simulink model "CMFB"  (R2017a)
settings: Solver=ode113  StartTime=0.0  StopTime=3  RelTol=1e-4  EnableMultiTasking=on
model workspace: external: MAT-File (data not in the file)
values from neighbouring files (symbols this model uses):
  Button = readtable('i_button.csv')    [CMFBoptimizer.m]
  Button_Stiffness = table(x_displacement,stiffness,activation_p,activation_d,activation_midair,damping)    [CMFBoptimizer.m]
  Finger = readtable('i_finger.csv')    [CMFBoptimizer.m]
  finger_start_height = random('norm',Finger.fstart_height,Finger.fstart_height_std)    [CMFBoptimizer.m]
  Finger_Stiffness = readtable('i_finger_stiffness.csv')    [CMFBoptimizer.m]
  Sensory = readtable('i_sensorynoise.csv')    [CMFBoptimizer.m]
undefined symbols (not defined in the file or in its folder): amplitude_ag, amplitude_an, b_penvel, Circle, circle_rad, Contact_Forces_Lib, deg, Extr_Data_Ring, Finite, Force, k_pen, kg, Law, Line, line_depth, line_length, m, max_out, min_out, N, PD, pen_exp, phasedelay_ag, PL, pulsewidth_ag, pulsewidth_an, PW, s, step_finish, step_start, to, vis_len_cirFx, vis_len_linBx, vis_len_linBz, vis_opc, vis_opc_en, window, X, Y, Z
libraries: nesl_utility x40, sm_lib x36, Contact_Forces_Lib x2, fl_lib x2, powerlib_meascontrol x1
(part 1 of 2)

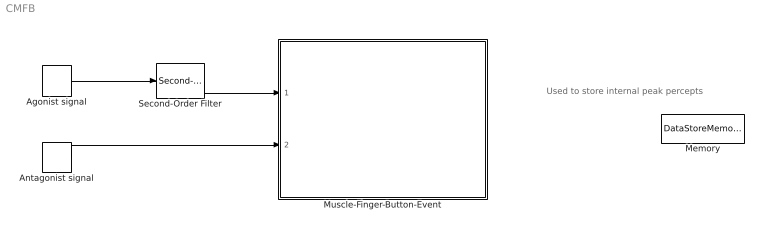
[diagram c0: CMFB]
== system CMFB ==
  note: Used to store internal peak percepts
  Agonist signal : DiscretePulseGenerator  PulseType=Time based  Amplitude=amplitude_ag  Period=window  PulseWidth=pulsewidth_ag  PhaseDelay=phasedelay_ag
  Antagonist signal : DiscretePulseGenerator  PulseType=Time based  Amplitude=amplitude_an  Period=window  PulseWidth=pulsewidth_an
  Memory : DataStoreMemory  DataStoreName=peak_int  ReadBeforeWriteMsg=warning  WriteAfterWriteMsg=warning  WriteAfterReadMsg=warning  InitialValue=0.1  ShowAdditionalParam=off  OutMin=0  OutMax=window
  Muscle-Finger-Button-Event : Subsystem
  Second-Order Filter : powerlib_meascontrol/Filters/Second-Order Filter  FilterType=Lowpass  Fo=4  Zeta=0.9  Ts=0  Initialize=on  Vac_Init="[0,  0,  60]"  Vdc_Init=0  PlotResponse=off  FreqRange=[0, 500, 1]
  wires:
  Antagonist signal/1 -> Muscle-Finger-Button-Event/2(Antagonist Muscle activation signal (0 to 1)1)
  Agonist signal/1 -> Second-Order Filter/1
  Second-Order Filter/1 -> Muscle-Finger-Button-Event/1(Agonist Muscle activation signal (0 to 1))

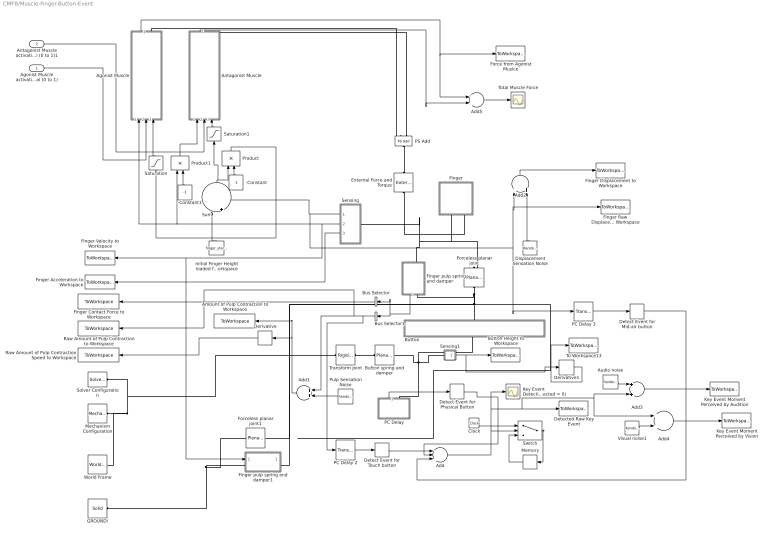
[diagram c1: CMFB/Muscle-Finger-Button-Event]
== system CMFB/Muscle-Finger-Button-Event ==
  Agonist Muscle activation signal (0 to 1) : Inport
  Antagonist Muscle activation signal (0 to 1)1 : Inport  Port=2
  -Constant : Constant  Value=-1
  -Constant1 : Constant  Value=-1
  Add : Sum  Inputs=+++
  Add{1..5} (5 alike) : Sum
  Agonist Muscle : Subsystem
  Amount of Pulp Contraction to Workspace : ToWorkspace  VariableName=pulpcontact  SaveFormat=Timeseries  SampleTime=-1
  Antagonist Muscle : Subsystem
  Audio noise : RandomNumber  Variance=Sensory.a_noise
  Bus Selector : BusSelector  OutputSignals=Normal Force  OutputAsBus=on
  Bus Selector1 : BusSelector  OutputSignals=Penetration  OutputAsBus=on
  Button : Subsystem  Tag=CustomStyle
  Button spring and damper : sm_lib/Joints/Planar Joint  SenseConstraintForce=off  SenseConstraintForceX=off  SenseConstraintForceY=off  SenseConstraintForceZ=off  SenseConstraintTorque=off  SenseConstraintTorqueX=off  SenseConstraintTorqueY=off  SenseConstraintTorqueZ=off  SenseTotalForce=off  SenseTotalForceX=off  SenseTotalForceY=off  SenseTotalForceZ=off  SenseTotalTorque=off  SenseTotalTorqueX=off  SenseTotalTorqueY=off  SenseTotalTorqueZ=off  CompositeWrenchDir=FollowerOnBase  CompositeWrenchFrame=BaseFrame  PxEquilibriumPosition=0  PxEquilibriumPositionUnits=m  PxSpringStiffness=0  PxSpringStiffnessUnits=N/m  PxDampingCoefficient=0  PxDampingCoefficientUnits=N/(m/s)  PxTorqueActuationMode=NoTorque  PxMotionActuationMode=ComputedMotion  PxSensePosition=off  PxSenseVelocity=off  PxSenseAcceleration=off  PxSenseTorqueForce=off  PxPositionTargetSpecify=off  PxPositionTargetPriority=High  PxPositionTargetValue=0  PxPositionTargetValueUnits=m  PxVelocityTargetSpecify=off  PxVelocityTargetPriority=High  PxVelocityTargetValue=0  PxVelocityTargetValueUnits=m/s  PyEquilibriumPosition=0  PyEquilibriumPositionUnits=m  PySpringStiffness=0  PySpringStiffnessUnits=N/m  PyDampingCoefficient=0  PyDampingCoefficientUnits=N/(m/s)  PyTorqueActuationMode=NoTorque  PyMotionActuationMode=ComputedMotion  PySensePosition=off  PySenseVelocity=off  PySenseAcceleration=off  PySenseTorqueForce=off  PyPositionTargetSpecify=off  PyPositionTargetPriority=High  PyPositionTargetValue=0  PyPositionTargetValueUnits=m  PyVelocityTargetSpecify=off  PyVelocityTargetPriority=High  PyVelocityTargetValue=0  PyVelocityTargetValueUnits=m/s  RzEquilibriumPosition=0  RzEquilibriumPositionUnits=deg  RzSpringStiffness=0  RzSpringStiffnessUnits=N*m/deg  RzDampingCoefficient=0  RzDampingCoefficientUnits=N*m/(deg/s)  RzTorqueActuationMode=NoTorque  RzMotionActuationMode=ComputedMotion  RzSensePosition=off  RzSenseVelocity=off  RzSenseAcceleration=off  RzSenseTorqueForce=off  RzPositionTargetSpecify=off  RzPositionTargetPriority=High  RzPositionTargetValue=0  RzPositionTargetValueUnits=deg  RzVelocityTargetSpecify=off  RzVelocityTargetPriority=High  RzVelocityTargetValue=0  RzVelocityTargetValueUnits=deg/s
  Button Height to Workspace : ToWorkspace  VariableName=buttonheight  SaveFormat=Timeseries  SampleTime=-1
  Clock : Clock
  Derivative : Derivative
  Derivative1 : Derivative
  Detect Event for Touch button : HitCross  HitCrossingOffset=Button_Stiffness.activation_p(1)  HitCrossingDirection=rising
  Detect Event for Physical Button : HitCross  HitCrossingOffset=Button_Stiffness.activation_d(1)  HitCrossingDirection=falling
  Detect Event for Mid-air button : HitCross  HitCrossingOffset=Button_Stiffness.activation_midair(1)  HitCrossingDirection=falling
  Detected Raw Key Event : ToWorkspace  VariableName=keyevent  SaveFormat=Timeseries  SampleTime=-1
  Displacement Sensation Noise : RandomNumber  Variance=Sensory.d_noise
  External Force and Torque : sm_lib/Forces and Torques/External Force and Torque  ForceResolutionFrame=World  EnableForceX=off  EnableForceY=off  EnableForceZ=on  EnableForce=off  TorqueResolutionFrame=AttachedFrame  EnableTorqueX=off  EnableTorqueY=off  EnableTorqueZ=off  EnableTorque=off
  Finger : Subsystem  Tag=CustomStyle
  Finger Acceleration to Workspace : ToWorkspace  VariableName=acceleration  SaveFormat=Timeseries  SampleTime=-1
  Finger Contact Force to Workspace : ToWorkspace  VariableName=raw_pulpcontact_force  SaveFormat=Timeseries  SampleTime=-1
  Finger Displacement to Workspace : ToWorkspace  VariableName=displacement  SaveFormat=Timeseries  SampleTime=-1
  Finger Raw Displacement to Workspace : ToWorkspace  VariableName=raw_displacement  SaveFormat=Timeseries  SampleTime=-1
  Finger Velocity to Workspace : ToWorkspace  VariableName=velocity  SaveFormat=Timeseries  SampleTime=-1
  Finger pulp spring and damper : Subsystem  AncestorBlock=Contact_Forces_Lib/2D/Circle to Finite Line Force
  Finger pulp spring and damper1 : Subsystem  AncestorBlock=Contact_Forces_Lib/2D/Circle to Finite Line Force
  Force from Agonist Muslce : ToWorkspace  VariableName=push_muscle_force  SaveFormat=Timeseries  SampleTime=-1
  Forceless planar joint : sm_lib/Joints/Planar Joint  SenseConstraintForce=off  SenseConstraintForceX=off  SenseConstraintForceY=off  SenseConstraintForceZ=off  SenseConstraintTorque=off  SenseConstraintTorqueX=off  SenseConstraintTorqueY=off  SenseConstraintTorqueZ=off  SenseTotalForce=off  SenseTotalForceX=off  SenseTotalForceY=off  SenseTotalForceZ=off  SenseTotalTorque=off  SenseTotalTorqueX=off  SenseTotalTorqueY=off  SenseTotalTorqueZ=off  CompositeWrenchDir=FollowerOnBase  CompositeWrenchFrame=BaseFrame  PxEquilibriumPosition=Finger.fstart_height  PxEquilibriumPositionUnits=m  PxSpringStiffness=0  PxSpringStiffnessUnits=N/m  PxDampingCoefficient=0  PxDampingCoefficientUnits=N/(m/s)  PxTorqueActuationMode=NoTorque  PxMotionActuationMode=ComputedMotion  PxSensePosition=off  PxSenseVelocity=off  PxSenseAcceleration=off  PxSenseTorqueForce=off  PxPositionTargetSpecify=on  PxPositionTargetPriority=High  PxPositionTargetValue=Finger.fstart_height  PxPositionTargetValueUnits=m  PxVelocityTargetSpecify=off  PxVelocityTargetPriority=High  PxVelocityTargetValue=-1  PxVelocityTargetValueUnits=m/s  PyEquilibriumPosition=0  PyEquilibriumPositionUnits=m  PySpringStiffness=0  PySpringStiffnessUnits=N/m  PyDampingCoefficient=0  PyDampingCoefficientUnits=N/(m/s)  PyTorqueActuationMode=NoTorque  PyMotionActuationMode=ComputedMotion  PySensePosition=off  PySenseVelocity=off  PySenseAcceleration=off  PySenseTorqueForce=off  PyPositionTargetSpecify=off  PyPositionTargetPriority=High  PyPositionTargetValue=0.49  PyPositionTargetValueUnits=m  PyVelocityTargetSpecify=off  PyVelocityTargetPriority=High  PyVelocityTargetValue=0  PyVelocityTargetValueUnits=m/s  RzEquilibriumPosition=0  RzEquilibriumPositionUnits=deg  RzSpringStiffness=0  RzSpringStiffnessUnits=N*m/deg  RzDampingCoefficient=0  RzDampingCoefficientUnits=N*m/(deg/s)  RzTorqueActuationMode=NoTorque  RzMotionActuationMode=ComputedMotion  RzSensePosition=off  RzSenseVelocity=off  RzSenseAcceleration=off  RzSenseTorqueForce=off  RzPositionTargetSpecify=off  RzPositionTargetPriority=High  RzPositionTargetValue=0  RzPositionTargetValueUnits=deg  RzVelocityTargetSpecify=off  RzVelocityTargetPriority=High  RzVelocityTargetValue=0  RzVelocityTargetValueUnits=deg/s
  Forceless planar joint1 : sm_lib/Joints/Planar Joint  SenseConstraintForce=off  SenseConstraintForceX=off  SenseConstraintForceY=off  SenseConstraintForceZ=off  SenseConstraintTorque=off  SenseConstraintTorqueX=off  SenseConstraintTorqueY=off  SenseConstraintTorqueZ=off  SenseTotalForce=off  SenseTotalForceX=off  SenseTotalForceY=off  SenseTotalForceZ=off  SenseTotalTorque=off  SenseTotalTorqueX=off  SenseTotalTorqueY=off  SenseTotalTorqueZ=off  CompositeWrenchDir=FollowerOnBase  CompositeWrenchFrame=BaseFrame  PxEquilibriumPosition=-Button.bdepth/2-Finger.fradius  PxEquilibriumPositionUnits=m  PxSpringStiffness=0  PxSpringStiffnessUnits=N/m  PxDampingCoefficient=Button_Stiffness.damping(1)  PxDampingCoefficientUnits=N/(m/s)  PxTorqueActuationMode=NoTorque  PxMotionActuationMode=ComputedMotion  PxSensePosition=off  PxSenseVelocity=off  PxSenseAcceleration=off  PxSenseTorqueForce=off  PxPositionTargetSpecify=on  PxPositionTargetPriority=High  PxPositionTargetValue=-Button.bdepth/2-Finger.fradius  PxPositionTargetValueUnits=m  PxVelocityTargetSpecify=off  PxVelocityTargetPriority=High  PxVelocityTargetValue=-1  PxVelocityTargetValueUnits=m/s  PyEquilibriumPosition=0  PyEquilibriumPositionUnits=m  PySpringStiffness=0  PySpringStiffnessUnits=N/m  PyDampingCoefficient=0  PyDampingCoefficientUnits=N/(m/s)  PyTorqueActuationMode=NoTorque  PyMotionActuationMode=ComputedMotion  PySensePosition=off  PySenseVelocity=off  PySenseAcceleration=off  PySenseTorqueForce=off  PyPositionTargetSpecify=off  PyPositionTargetPriority=High  PyPositionTargetValue=0.49  PyPositionTargetValueUnits=m  PyVelocityTargetSpecify=off  PyVelocityTargetPriority=High  PyVelocityTargetValue=0  PyVelocityTargetValueUnits=m/s  RzEquilibriumPosition=0  RzEquilibriumPositionUnits=deg  RzSpringStiffness=0  RzSpringStiffnessUnits=N*m/deg  RzDampingCoefficient=0  RzDampingCoefficientUnits=N*m/(deg/s)  RzTorqueActuationMode=NoTorque  RzMotionActuationMode=ComputedMotion  RzSensePosition=off  RzSenseVelocity=off  RzSenseAcceleration=off  RzSenseTorqueForce=off  RzPositionTargetSpecify=off  RzPositionTargetPriority=High  RzPositionTargetValue=0  RzPositionTargetValueUnits=deg  RzVelocityTargetSpecify=off  RzVelocityTargetPriority=High  RzVelocityTargetValue=0  RzVelocityTargetValueUnits=deg/s
  GROUND! : sm_lib/Body Elements/Solid  InertiaType=CalculateFromGeometry  Mass=1  MassUnits=kg  CenterOfMass=[0 0 0]  CenterOfMassUnits=m  MomentsOfInertia=[1 1 1]  MomentsOfInertiaUnits=kg*m^2  ProductsOfInertia=[1 1 1]  ProductsOfInertiaUnits=kg*m^2  DensityBased=on  Density=99999999999999  DensityUnits=kg/m^3  DoExposeReferenceFrame=on  SerializedFrames=<Frames/>  GraphicType=None  MarkerShape=Sphere  MarkerSize=10  GraphicVisPropType=SimpleVisualProperties  GraphicDiffuseColor=[0.5 0.5 0.5]  GraphicSpecularColor=[0.5 0.5 0.5 1.0]  GraphicAmbientColor=[0.15 0.15 0.15 1.0]  GraphicEmissiveColor=[0.0 0.0 0.0 1.0]  GraphicShininess=75  GraphicOpacity=1.0  GeometryShape=Sphere  RectangleSize=[1 1]  RectangleSizeUnits=m  BrickDimensions=[1 1 1]  BrickDimensionUnits=m  CylinderRadius=1  CylinderRadiusUnits=m  CylinderLength=1  CylinderLengthUnits=m  SphereRadius=Finger.fradius  SphereRadiusUnits=m  EllipsoidRadii=[1 1 1]  EllipsoidRadiiUnits=m  ExtrusionCrossSection=[1 1; -1 1; -1 -1; 1 -1]  ExtrusionCrossSectionUnits=m  ExtrusionLength=1  ExtrusionLengthUnits=m  PolygonNumSides=3  PolygonOuterRadius=1  PolygonOuterRadiusUnits=m  ExtGeomFileType=STEP  ExtGeomFileUnits=m  RevolutionCrossSection=[1 1; 1 -1; 2 -1; 2 1]  RevolutionCrossSectionUnits=m  RevolutionExtent=Full  RevolutionAngle=180  RevolutionAngleUnits=deg
  Initial Finger Height loaded from Workspace : Constant  Value=finger_start_height
  "Key Event Detection (detected = 1, not detected = 0)" : Scope
  Key Event Moment Perceived by Audition : ToWorkspace  VariableName=keyeventtime_a  SaveFormat=Timeseries  SampleTime=-1
  Key Event Moment Perceived by Vision : ToWorkspace  VariableName=keyeventtime_l  SaveFormat=Timeseries  SampleTime=-1
  Mechanism Configuration : sm_lib/Utilities/Mechanism Configuration  UniformGravity=None  GravityVector=[0 0 0]  GravityUnits=m/s^2  LinearizationDelta=0.001
  Memory : Memory
  PC Delay : Subsystem
  PC Delay 2 : TransportDelay  DelayTime=Button.bea_delay
  PC Delay 3 : TransportDelay  DelayTime=Button.bea_delay
  PS Add : fl_lib/Physical Signals/Functions/PS Add
  Product : Product
  Product1 : Product
  Pulp Sensation Noise : RandomNumber  Variance=Sensory.p_noise
  Raw Amount of Pulp Contraction Speed to Workspace : ToWorkspace  VariableName=pulpcontact_derivate  SaveFormat=Timeseries  SampleTime=-1
  Raw Amount of Pulp Contraction to Workspace : ToWorkspace  VariableName=raw_pulpcontact  SaveFormat=Timeseries  SampleTime=-1
  Saturation : Saturate  UpperLimit=Finger.Lmag  LowerLimit=-Finger.Lmag
  Saturation1 : Saturate  UpperLimit=Finger.Lman  LowerLimit=-Finger.Lman
  Sensing : Subsystem
  Sensing1 : Subsystem
  Solver Configuration : nesl_utility/Solver Configuration  PhysicalDomain=network_engine_domain  SubClassName=solver  LeftPortType=input  RightPortType=generic  Accelerate=off  Tones=[]  Harmonics=[]  SimulateNoise=off  Profile=off  UseLocalSampling=off  EnableSwitchedLinearOptims=on  FrequencyDomain=off  UseCCode=off  RelTol=0.001  AbsTol=1e-06  MinStep=1e-09  ToWorkspace=off  RevertToSquareIcSolve=off  NumHomotopyIterations=100  PhasorMode=off  PhasorModeNumHarmonics=1  OverrideAbsTol=off  DoDC=off  ResidualTolerance=1e-9  UseLocalSolver=off  LocalSolverChoice=NE_TRAPEZOIDAL_ADVANCER  LocalSolverSampleTime=.0001  DoFixedCost=off  MaxNonlinIter=3  MaxModeIter=2  LinearAlgebra=Sparse  DelaysMemoryBudget=1024  AutomaticFiltering=on  FilteringTimeConstant=0.001
  Sum : Sum  Inputs=|+-
  Switch : Switch  Criteria=u2 > Threshold
  To Workspace13 : ToWorkspace  VariableName=buttonvelocity  SaveFormat=Timeseries  SampleTime=-1
  Total Muscle Force : Scope
  Transform Joint : sm_lib/Frames and Transforms/Rigid Transform  TranslationMethod=None  TranslationStandardOffset=0  TranslationLengthUnit=m  TranslationStandardAxis=+Z  TranslationCartesianOffset=[0 0 0]  TranslationROffset=0  TranslationROffsetUnits=m  TranslationZOffset=0  TranslationZOffsetUnits=m  TranslationThetaOffset=0  TranslationThetaOffsetUnits=deg  RotationMethod=StandardAxis  RotationAngleUnits=deg  RotationStandardAxis=+X  RotationAngle=90  RotationArbitraryAxis=[0 0 1]  FollAlignAxisA=+X  BaseAlignAxisA=+Y  FollAlignAxisB=+Y  BaseAlignAxisB=+Z  RotationSequenceAxes=FollowerAxes  RotationSequence=XYX  RotationSequenceAngles=[0 0 0]  RotationSequenceAnglesUnits=deg  RotationMatrix=[1 0 0; 0 1 0; 0 0 1]
  Visual noise1 : RandomNumber  Variance=Sensory.l_noise
  World Frame : sm_lib/Frames and Transforms/World Frame
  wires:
  Antagonist Muscle/1(Muscle force (S)) -> Add5/2
  Sensing/3(A) -> Finger Acceleration to Workspace/1
  Initial Finger Height loaded from Workspace/1 -> Sum/1
  Bus Selector/1 -> Finger Contact Force to Workspace/1
  Sensing1/1(S) -> Derivative1/1, Button Height to Workspace/1
  Sensing/1(P) -> PC Delay 3/1, Finger Raw Displacement to Workspace/1, Add2/1, Sum/2
  PC Delay/1(S) -> Detect Event for Physical Button/1
  Finger pulp spring and damper/1(Out) -> Bus Selector/1, Bus Selector1/1
  Detect Event for Physical Button/1 -> Add/2
  Clock/1 -> Switch/1
  Switch/1 -> Memory/1
  Memory/1 -> Switch/3
  Agonist Muscle/1(Muscle force (S)) -> Force from Agonist Muslce/1, Add5/1
  Sum/1 -> Saturation1/1, Product/1
  -Constant/1 -> Product/2
  Product1/1 -> Antagonist Muscle/1(Muscle Velocity)
  -Constant1/1 -> Product1/2
  Agonist Muscle activation signal (0 to 1)/1 -> Agonist Muscle/2(Muscle Activation Level)
  Antagonist Muscle activation signal (0 to 1)1/1 -> Antagonist Muscle/2(Muscle Activation Level)
  Saturation/1 -> Agonist Muscle/3(Muscle Strain)
  Saturation1/1 -> Antagonist Muscle/3(Muscle Strain)
  Product/1 -> Saturation/1
  Derivative/1 -> Raw Amount of Pulp Contraction Speed to Workspace/1
  Bus Selector1/1 -> PC Delay 2/1, Raw Amount of Pulp Contraction to Workspace/1, Add1/1
  Add/1 -> Switch/2, Add4/1, Add3/2, Detected Raw Key Event/1, "Key Event Detection (detected = 1, not detected = 0)"/1
  Detect Event for Touch button/1 -> Add/1
  PC Delay 2/1 -> Detect Event for Touch button/1
  Pulp Sensation Noise/1 -> Add1/2
  Add1/1 -> Amount of Pulp Contraction to Workspace/1, Derivative/1
  Displacement Sensation Noise/1 -> Add2/2
  Add2/1 -> Finger Displacement to Workspace/1
  Audio noise/1 -> Add3/1
  Add3/1 -> Key Event Moment Perceived by Audition/1
  Visual noise1/1 -> Add4/2
  Add4/1 -> Key Event Moment Perceived by Vision/1
  PC Delay 3/1 -> Detect Event for Mid-air button/1
  Detect Event for Mid-air button/1 -> Add/3
  Add5/1 -> Total Muscle Force/1
  Derivative1/1 -> To Workspace13/1
  Sensing/2(V) -> Finger pulp spring and damper1/1(fv), Finger Velocity to Workspace/1, Product1/1, Agonist Muscle/1(Muscle Velocity)
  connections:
  Forceless planar joint/LConn1 -- Finger pulp spring and damper1/RConn1 -- Forceless planar joint1/LConn1 -- Finger pulp spring and damper/RConn1 -- Button/RConn1
  Finger/RConn1 -- Forceless planar joint/RConn1 -- Sensing/LConn1 -- Finger pulp spring and damper/LConn1
  PC Delay/RConn1 -- Button spring and damper/RConn1 -- Sensing1/LConn1 -- Button/LConn1
  Transform Joint/LConn1 -- World Frame/RConn1 -- Mechanism Configuration/RConn1 -- Solver Configuration/RConn1
  External Force and Torque/RConn1 -- Finger/RConn2
  Transform Joint/RConn1 -- Button spring and damper/LConn1
  Agonist Muscle/RConn1 -- PS Add/LConn2
  PS Add/RConn1 -- External Force and Torque/LConn1
  Antagonist Muscle/RConn1 -- PS Add/LConn1
  GROUND!/RConn1 -- Finger pulp spring and damper1/LConn1 -- Forceless planar joint1/RConn1

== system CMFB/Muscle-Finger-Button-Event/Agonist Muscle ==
  Muscle Velocity : Inport
  Muscle Activation Level : Inport  Port=2
  Muscle Strain : Inport  Port=3
  "  1" : Constant  Value=Finger.fcsa
  "  3" : Constant  Value=0
  Fce : Product  Inputs=3
  MinMax1 : MinMax  Inputs=2
  MinMax2 : MinMax  Function=max  Inputs=2
  MinMax3 : MinMax  Function=max  Inputs=2
  Mux2 : Mux  Inputs=2
  Scope : Scope
  Simulink-PS Converter : nesl_utility/Simulink-PS Converter  PhysicalDomain=network_engine_domain  SubClassName=ps_input  LeftPortType=input  RightPortType=output  PseudoPeriodic=off  Frequencies=[]  NoiseDistribution=none  NoiseParameters=[]  Unit=1  AffineConversion=off  FilteringAndDerivatives=zero  SimscapeFilterOrder=1  InputFilterTimeConstant=0.001  UdotUserProvided=1
  Sum : Sum  Inputs=|--
  fp : Fcn  Expr=Finger.Ks*(exp(Finger.Kc*u(1)/Finger.L0ag)-1)+Finger.Kd*u(2)/Finger.L0ag
  fv : Fcn  Expr=1+u/Finger.vmag
  Muscle Force : PMIOPort  Port=1  Side=Right
  Muscle force (S) : Outport
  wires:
  Muscle Strain/1 -> Mux2/1
  Muscle Velocity/1 -> MinMax1/1, Mux2/2
  Mux2/1 -> fp/1
  fp/1 -> MinMax2/1
  "  3"/1 -> MinMax1/2, MinMax3/2, MinMax2/2
  MinMax1/1 -> fv/1
  fv/1 -> MinMax3/1
  Muscle Activation Level/1 -> Fce/1
  MinMax3/1 -> Fce/3
  "  1"/1 -> Fce/2
  Fce/1 -> Sum/1
  MinMax2/1 -> Scope/1, Sum/2
  Sum/1 -> Muscle force (S)/1, Simulink-PS Converter/1
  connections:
  Muscle Force/RConn1 -- Simulink-PS Converter/RConn1

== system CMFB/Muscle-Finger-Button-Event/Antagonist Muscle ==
  Muscle Velocity : Inport
  Muscle Activation Level : Inport  Port=2
  Muscle Strain : Inport  Port=3
  "  1" : Constant  Value=Finger.fcsa
  "  3" : Constant  Value=0
  Fce : Product  Inputs=3
  MinMax1 : MinMax  Inputs=2
  MinMax2 : MinMax  Function=max  Inputs=2
  MinMax3 : MinMax  Function=max  Inputs=2
  Mux2 : Mux  Inputs=2
  Simulink-PS Converter : nesl_utility/Simulink-PS Converter  PhysicalDomain=network_engine_domain  SubClassName=ps_input  LeftPortType=input  RightPortType=output  PseudoPeriodic=off  Frequencies=[]  NoiseDistribution=none  NoiseParameters=[]  Unit=1  AffineConversion=off  FilteringAndDerivatives=zero  SimscapeFilterOrder=1  InputFilterTimeConstant=0.001  UdotUserProvided=1
  Sum : Sum  Inputs=|++
  fp : Fcn  Expr=Finger.Ks*(exp(Finger.Kc*u(1)/Finger.L0an)-1)+Finger.Kd*u(2)/Finger.L0an
  fv : Fcn  Expr=1+u/Finger.vman
  Muscle Force : PMIOPort  Port=1  Side=Right
  Muscle force (S) : Outport
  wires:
  Muscle Strain/1 -> Mux2/1
  Muscle Velocity/1 -> MinMax1/1, Mux2/2
  Mux2/1 -> fp/1
  fp/1 -> MinMax2/1
  "  3"/1 -> MinMax1/2, MinMax3/2, MinMax2/2
  MinMax1/1 -> fv/1
  fv/1 -> MinMax3/1
  Muscle Activation Level/1 -> Fce/1
  MinMax3/1 -> Fce/3
  "  1"/1 -> Fce/2
  Fce/1 -> Sum/1
  MinMax2/1 -> Sum/2
  Sum/1 -> Muscle force (S)/1, Simulink-PS Converter/1
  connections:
  Muscle Force/RConn1 -- Simulink-PS Converter/RConn1

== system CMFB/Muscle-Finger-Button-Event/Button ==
  Button : sm_lib/Body Elements/Solid  InertiaType=CalculateFromGeometry  Mass=1  MassUnits=kg  CenterOfMass=[0 0 0]  CenterOfMassUnits=m  MomentsOfInertia=[1 1 1]  MomentsOfInertiaUnits=kg*m^2  ProductsOfInertia=[0 0 0]  ProductsOfInertiaUnits=kg*m^2  DensityBased=on  Density=P_rho  DensityUnits=kg/(m^3)  DoExposeReferenceFrame=on  SerializedFrames=<Frames/>  GraphicType=FromGeometry  MarkerShape=Sphere  MarkerSize=10  MarkerSizeUnits=m  GraphicVisPropType=SimpleVisualProperties  GraphicDiffuseColor=[0 0.6 0]  GraphicSpecularColor=[0.5 0.5 0.5 1.0]  GraphicAmbientColor=[0.15 0.15 0.15 1.0]  GraphicEmissiveColor=[0.0 0.0 0.0 1.0]  GraphicShininess=75  GraphicOpacity=1.0  GeometryShape=Brick  RectangleSize=[1 1]  RectangleSizeUnits=m  BrickDimensions=[PL PW PD]  BrickDimensionUnits=m  CylinderRadius=1  CylinderRadiusUnits=m  CylinderLength=1  CylinderLengthUnits=m  SphereRadius=1  SphereRadiusUnits=m  EllipsoidRadii=[1 1 1]  EllipsoidRadiiUnits=m  ExtrusionCrossSection=[1 1; -1 1; -1 -1; 1 -1]  ExtrusionCrossSectionUnits=m  ExtrusionLength=1  ExtrusionLengthUnits=m  PolygonNumSides=3  PolygonOuterRadius=1  PolygonOuterRadiusUnits=m  ExtGeomFileType=STL  ExtGeomFileUnits=m  RevolutionCrossSection=[1 1; 1 -1; 2 -1; 2 1]  RevolutionCrossSectionUnits=m  RevolutionExtent=Full  RevolutionAngle=180  RevolutionAngleUnits=deg
  Transform Button : sm_lib/Frames and Transforms/Rigid Transform  TranslationMethod=None  TranslationStandardOffset=0  TranslationLengthUnit=m  TranslationStandardAxis=+Z  TranslationCartesianOffset=[0 0 0]  TranslationROffset=0  TranslationROffsetUnits=m  TranslationZOffset=0  TranslationZOffsetUnits=m  TranslationThetaOffset=0  TranslationThetaOffsetUnits=deg  RotationMethod=StandardAxis  RotationAngleUnits=deg  RotationStandardAxis=+X  RotationAngle=90  RotationArbitraryAxis=[0 0 1]  FollAlignAxisA=+X  BaseAlignAxisA=+Y  FollAlignAxisB=+Y  BaseAlignAxisB=+Z  RotationSequenceAxes=FollowerAxes  RotationSequence=XYX  RotationSequenceAngles=[0 0 0]  RotationSequenceAnglesUnits=deg  RotationMatrix=[1 0 0; 0 1 0; 0 0 1]
  Transform Pulp : sm_lib/Frames and Transforms/Rigid Transform  TranslationMethod=None  TranslationStandardOffset=0  TranslationLengthUnit=m  TranslationStandardAxis=+Z  TranslationCartesianOffset=[0 0 0]  TranslationROffset=0  TranslationROffsetUnits=m  TranslationZOffset=0  TranslationZOffsetUnits=m  TranslationThetaOffset=0  TranslationThetaOffsetUnits=deg  RotationMethod=AlignedAxes  RotationAngleUnits=deg  RotationStandardAxis=+Z  RotationAngle=0  RotationArbitraryAxis=[0 0 1]  FollAlignAxisA=+X  BaseAlignAxisA=+Z  FollAlignAxisB=+Y  BaseAlignAxisB=+X  RotationSequenceAxes=FollowerAxes  RotationSequence=XYX  RotationSequenceAngles=[0 0 0]  RotationSequenceAnglesUnits=deg  RotationMatrix=[1 0 0; 0 1 0; 0 0 1]
  B : PMIOPort  Port=1  Side=Right
  P : PMIOPort  Port=2  Side=Left
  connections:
  Transform Button/RConn1 -- P/RConn1
  Button/RConn1 -- Transform Button/LConn1 -- Transform Pulp/LConn1
  Transform Pulp/RConn1 -- B/RConn1

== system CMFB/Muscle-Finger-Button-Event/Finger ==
  Finger : sm_lib/Body Elements/Solid  InertiaType=CalculateFromGeometry  Mass=1  MassUnits=kg  CenterOfMass=[0 0 0]  CenterOfMassUnits=m  MomentsOfInertia=[1 1 1]  MomentsOfInertiaUnits=kg*m^2  ProductsOfInertia=[0 0 0]  ProductsOfInertiaUnits=kg*m^2  DensityBased=on  Density=F_rho  DensityUnits=kg/(m^3)  DoExposeReferenceFrame=on  SerializedFrames=<Frames/>  GraphicType=FromGeometry  MarkerShape=Sphere  MarkerSize=10  MarkerSizeUnits=m  GraphicVisPropType=SimpleVisualProperties  GraphicDiffuseColor=[0.6 0.0 0.0]  GraphicSpecularColor=[0.5 0.5 0.5 1.0]  GraphicAmbientColor=[0.15 0.15 0.15 1.0]  GraphicEmissiveColor=[0.0 0.0 0.0 1.0]  GraphicShininess=75  GraphicOpacity=1.0  GeometryShape=Cylinder  RectangleSize=[1 1]  RectangleSizeUnits=m  BrickDimensions=[0.5 0.5 0.05]  BrickDimensionUnits=m  CylinderRadius=FR  CylinderRadiusUnits=m  CylinderLength=FL  CylinderLengthUnits=m  SphereRadius=1  SphereRadiusUnits=m  EllipsoidRadii=[1 1 1]  EllipsoidRadiiUnits=m  ExtrusionCrossSection=[1 1; -1 1; -1 -1; 1 -1]  ExtrusionCrossSectionUnits=m  ExtrusionLength=1  ExtrusionLengthUnits=m  PolygonNumSides=3  PolygonOuterRadius=1  PolygonOuterRadiusUnits=m  ExtGeomFileType=STL  ExtGeomFileUnits=m  RevolutionCrossSection=[1 1; 1 -1; 2 -1; 2 1]  RevolutionCrossSectionUnits=m  RevolutionExtent=Full  RevolutionAngle=180  RevolutionAngleUnits=deg
  R : PMIOPort  Port=1  Side=Right
  R1 : PMIOPort  Port=2  Side=Right
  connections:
  Finger/RConn1 -- R1/RConn1 -- R/RConn1

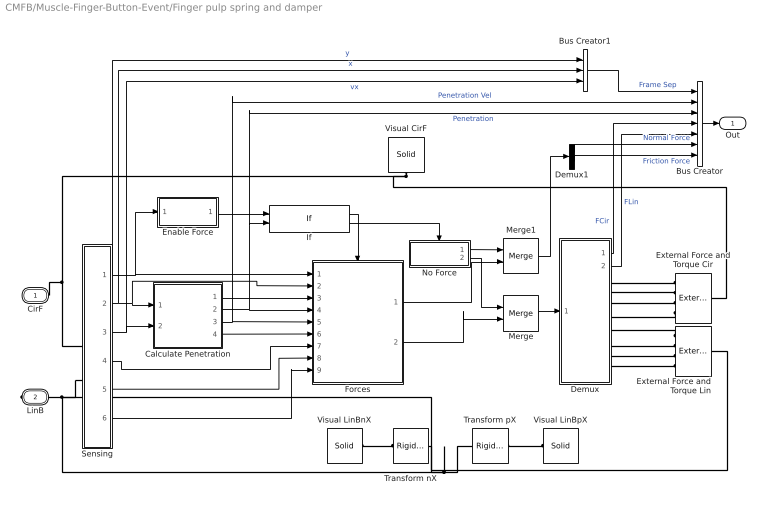
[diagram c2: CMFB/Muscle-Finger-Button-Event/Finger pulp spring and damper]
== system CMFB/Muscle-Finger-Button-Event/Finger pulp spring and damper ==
  Bus Creator : BusCreator  Inputs=7
  Bus Creator1 : BusCreator  Inputs=3
  Calculate Penetration : Subsystem
  Demux : Subsystem
  Demux1 : Demux  Outputs=2
  Enable Force : Subsystem
  External Force and Torque Cir : sm_lib/Forces and Torques/External Force and Torque  ForceResolutionFrame=AttachedFrame  EnableForceX=on  EnableForceY=on  EnableForceZ=on  EnableForce=off  TorqueResolutionFrame=AttachedFrame  EnableTorqueX=off  EnableTorqueY=off  EnableTorqueZ=on  EnableTorque=off
  External Force and Torque Lin : sm_lib/Forces and Torques/External Force and Torque  ForceResolutionFrame=AttachedFrame  EnableForceX=on  EnableForceY=on  EnableForceZ=on  EnableForce=off  TorqueResolutionFrame=AttachedFrame  EnableTorqueX=off  EnableTorqueY=off  EnableTorqueZ=on  EnableTorque=off
  Forces : Subsystem
  If : If  NumInputs=2  IfExpression=(u1 > 0 & u2>0)
  Merge : Merge  InitialOutput=0  InputPortOffsets=0
  Merge1 : Merge  InitialOutput=0  InputPortOffsets=0
  No Force : Subsystem
  Sensing : Subsystem
  Transform nX : sm_lib/Frames and Transforms/Rigid Transform  TranslationMethod=StandardAxis  TranslationStandardOffset=line_depth-vis_len_linBx/2  TranslationLengthUnit=m  TranslationStandardAxis=-X  TranslationCartesianOffset=[0 0 0]  TranslationROffset=0  TranslationROffsetUnits=m  TranslationZOffset=0  TranslationZOffsetUnits=m  TranslationThetaOffset=0  TranslationThetaOffsetUnits=deg  RotationMethod=None  RotationAngleUnits=deg  RotationStandardAxis=+Z  RotationAngle=0.0  RotationArbitraryAxis=[0 0 1]  FollAlignAxisA=+X  BaseAlignAxisA=+Y  FollAlignAxisB=+Y  BaseAlignAxisB=+Z  RotationSequenceAxes=FollowerAxes  RotationSequence=XYX  RotationSequenceAngles=[0 0 0]  RotationSequenceAnglesUnits=deg  RotationMatrix=[1 0 0; 0 1 0; 0 0 1]
  Transform pX : sm_lib/Frames and Transforms/Rigid Transform  TranslationMethod=StandardAxis  TranslationStandardOffset=line_depth-vis_len_linBx/2  TranslationLengthUnit=m  TranslationStandardAxis=+X  TranslationCartesianOffset=[0 0 0]  TranslationROffset=0  TranslationROffsetUnits=m  TranslationZOffset=0  TranslationZOffsetUnits=m  TranslationThetaOffset=0  TranslationThetaOffsetUnits=deg  RotationMethod=None  RotationAngleUnits=deg  RotationStandardAxis=+Z  RotationAngle=0.0  RotationArbitraryAxis=[0 0 1]  FollAlignAxisA=+X  BaseAlignAxisA=+Y  FollAlignAxisB=+Y  BaseAlignAxisB=+Z  RotationSequenceAxes=FollowerAxes  RotationSequence=XYX  RotationSequenceAngles=[0 0 0]  RotationSequenceAnglesUnits=deg  RotationMatrix=[1 0 0; 0 1 0; 0 0 1]
  Visual CirF : sm_lib/Body Elements/Solid  InertiaType=CalculateFromGeometry  Mass=1  MassUnits=kg  CenterOfMass=[0 0 0]  CenterOfMassUnits=m  MomentsOfInertia=[1 1 1]  MomentsOfInertiaUnits=kg*m^2  ProductsOfInertia=[0 0 0]  ProductsOfInertiaUnits=kg*m^2  DensityBased=on  Density=0  DensityUnits=kg/(m^3)  DoExposeReferenceFrame=on  SerializedFrames=<Frames/>  GraphicType=FromGeometry  MarkerShape=Sphere  MarkerSize=10  GraphicVisPropType=SimpleVisualProperties  GraphicDiffuseColor=vis_clr  GraphicSpecularColor=[0.5 0.5 0.5 1.0]  GraphicAmbientColor=[0.15 0.15 0.15 1.0]  GraphicEmissiveColor=[0.0 0.0 0.0 1.0]  GraphicShininess=75  GraphicOpacity=vis_opc*vis_opc_en  GeometryShape=GeneralExtrusion  RectangleSize=[1 1]  RectangleSizeUnits=m  BrickDimensions=[1 1 1]  BrickDimensionUnits=m  CylinderRadius=1  CylinderRadiusUnits=m  CylinderLength=1  CylinderLengthUnits=m  SphereRadius=1  SphereRadiusUnits=m  EllipsoidRadii=[1 1 1]  EllipsoidRadiiUnits=m  ExtrusionCrossSection=Extr_Data_Ring(circle_rad,circle_rad-vis_len_cirFx,0,360)  ExtrusionCrossSectionUnits=m  ExtrusionLength=vis_len_cirFz  ExtrusionLengthUnits=m  PolygonNumSides=3  PolygonOuterRadius=1  PolygonOuterRadiusUnits=m  ExtGeomFileType=STEP  ExtGeomFileUnits=m  RevolutionCrossSection=[1 1; 1 -1; 2 -1; 2 1]  RevolutionCrossSectionUnits=m  RevolutionExtent=Full  RevolutionAngle=180  RevolutionAngleUnits=deg
  Visual LinBnX : sm_lib/Body Elements/Solid  InertiaType=CalculateFromGeometry  Mass=1  MassUnits=kg  CenterOfMass=[0 0 0]  CenterOfMassUnits=m  MomentsOfInertia=[1 1 1]  MomentsOfInertiaUnits=kg*m^2  ProductsOfInertia=[0 0 0]  ProductsOfInertiaUnits=kg*m^2  DensityBased=on  Density=0  DensityUnits=kg/(m^3)  DoExposeReferenceFrame=on  SerializedFrames=<Frames/>  GraphicType=FromGeometry  MarkerShape=Sphere  MarkerSize=10  GraphicVisPropType=SimpleVisualProperties  GraphicDiffuseColor=vis_clr  GraphicSpecularColor=[0.5 0.5 0.5 1.0]  GraphicAmbientColor=[0.15 0.15 0.15 1.0]  GraphicEmissiveColor=[0.0 0.0 0.0 1.0]  GraphicShininess=75  GraphicOpacity=vis_opc*vis_opc_en  GeometryShape=Brick  RectangleSize=[1 1]  RectangleSizeUnits=m  BrickDimensions=[vis_len_linBx line_length vis_len_linBz]  BrickDimensionUnits=m  CylinderRadius=1  CylinderRadiusUnits=m  CylinderLength=1  CylinderLengthUnits=m  SphereRadius=1  SphereRadiusUnits=m  EllipsoidRadii=[1 1 1]  EllipsoidRadiiUnits=m  ExtrusionCrossSection=[1 1; -1 1; -1 -1; 1 -1]  ExtrusionCrossSectionUnits=m  ExtrusionLength=1  ExtrusionLengthUnits=m  PolygonNumSides=3  PolygonOuterRadius=1  PolygonOuterRadiusUnits=m  ExtGeomFileType=STEP  ExtGeomFileUnits=m  RevolutionCrossSection=[1 1; 1 -1; 2 -1; 2 1]  RevolutionCrossSectionUnits=m  RevolutionExtent=Full  RevolutionAngle=180  RevolutionAngleUnits=deg
  Visual LinBpX : sm_lib/Body Elements/Solid  InertiaType=CalculateFromGeometry  Mass=1  MassUnits=kg  CenterOfMass=[0 0 0]  CenterOfMassUnits=m  MomentsOfInertia=[1 1 1]  MomentsOfInertiaUnits=kg*m^2  ProductsOfInertia=[0 0 0]  ProductsOfInertiaUnits=kg*m^2  DensityBased=on  Density=0  DensityUnits=kg/(m^3)  DoExposeReferenceFrame=on  SerializedFrames=<Frames/>  GraphicType=FromGeometry  MarkerShape=Sphere  MarkerSize=10  GraphicVisPropType=SimpleVisualProperties  GraphicDiffuseColor=vis_clr  GraphicSpecularColor=[0.5 0.5 0.5 1.0]  GraphicAmbientColor=[0.15 0.15 0.15 1.0]  GraphicEmissiveColor=[0.0 0.0 0.0 1.0]  GraphicShininess=75  GraphicOpacity=vis_opc*vis_opc_en  GeometryShape=Brick  RectangleSize=[1 1]  RectangleSizeUnits=m  BrickDimensions=[vis_len_linBx line_length vis_len_linBz]  BrickDimensionUnits=m  CylinderRadius=1  CylinderRadiusUnits=m  CylinderLength=1  CylinderLengthUnits=m  SphereRadius=1  SphereRadiusUnits=m  EllipsoidRadii=[1 1 1]  EllipsoidRadiiUnits=m  ExtrusionCrossSection=[1 1; -1 1; -1 -1; 1 -1]  ExtrusionCrossSectionUnits=m  ExtrusionLength=1  ExtrusionLengthUnits=m  PolygonNumSides=3  PolygonOuterRadius=1  PolygonOuterRadiusUnits=m  ExtGeomFileType=STEP  ExtGeomFileUnits=m  RevolutionCrossSection=[1 1; 1 -1; 2 -1; 2 1]  RevolutionCrossSectionUnits=m  RevolutionExtent=Full  RevolutionAngle=180  RevolutionAngleUnits=deg
  CirF : PMIOPort  Tag=PMCPort  Port=1  Side=Left
  LinB : PMIOPort  Tag=PMCPort  Port=2  Side=Right
  Out : Outport
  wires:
  Merge1/1 -> Demux1/1
  Forces/1(Fnf) -> Merge1/2
  No Force/1(Fnf) -> Merge1/1
  Demux1/2 -> Bus Creator/7  "Friction Force"
  Demux1/1 -> Bus Creator/6  "Normal Force"
  Bus Creator1/1 -> Bus Creator/1  "Frame Sep"
  Bus Creator/1 -> Out/1
  Demux/1(FCir) -> Bus Creator/4  "FCir"
  Demux/2(FLin) -> Bus Creator/5  "FLin"
  Sensing/2(x) -> Bus Creator1/2, Forces/2(X Sep), Calculate Penetration/1(x)  "x"
  Sensing/3(vx) -> Calculate Penetration/2(vx), Bus Creator1/3  "vx"
  Calculate Penetration/4(Vel Sign) -> Forces/6(Vel_Cmp)
  Calculate Penetration/1(Pos Sign) -> Forces/3(Pos Cmp)
  Sensing/1(y) -> Bus Creator1/1, Enable Force/1(y), Forces/1(M arm)  "y"
  Calculate Penetration/2(Pen) -> If/2, Bus Creator/3, Forces/4(Pen)  "Penetration"
  Enable Force/1(Enable) -> If/1
  If/1 -> Forces/Action
  No Force/2(F) -> Merge/1
  If/2 -> No Force/Action
  Merge/1 -> Demux/1(F)
  Calculate Penetration/3(Pen Vel) -> Forces/5(Vel), Bus Creator/2  "Penetration Vel"
  Sensing/4(q) -> Forces/7(Unit Vector)
  Forces/2(F) -> Merge/2
  Sensing/5(vy) -> Forces/8(vy)
  Sensing/6(wz) -> Forces/9(wz)
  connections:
  Transform nX/RConn1 -- Visual LinBnX/RConn1
  Transform pX/RConn1 -- Visual LinBpX/RConn1
  Sensing/LConn2 -- External Force and Torque Lin/RConn1 -- Transform pX/LConn1 -- Transform nX/LConn1 -- LinB/RConn1
  Visual CirF/RConn1 -- Sensing/LConn1 -- CirF/RConn1 -- External Force and Torque Cir/RConn1
  Demux/RConn1 -- External Force and Torque Cir/LConn1
  External Force and Torque Cir/LConn2 -- Demux/RConn2
  Demux/RConn3 -- External Force and Torque Cir/LConn3
  External Force and Torque Lin/LConn1 -- Demux/RConn5
  Demux/RConn6 -- External Force and Torque Lin/LConn2
  External Force and Torque Lin/LConn3 -- Demux/RConn7
  Demux/RConn8 -- External Force and Torque Lin/LConn4
  External Force and Torque Cir/LConn4 -- Demux/RConn4

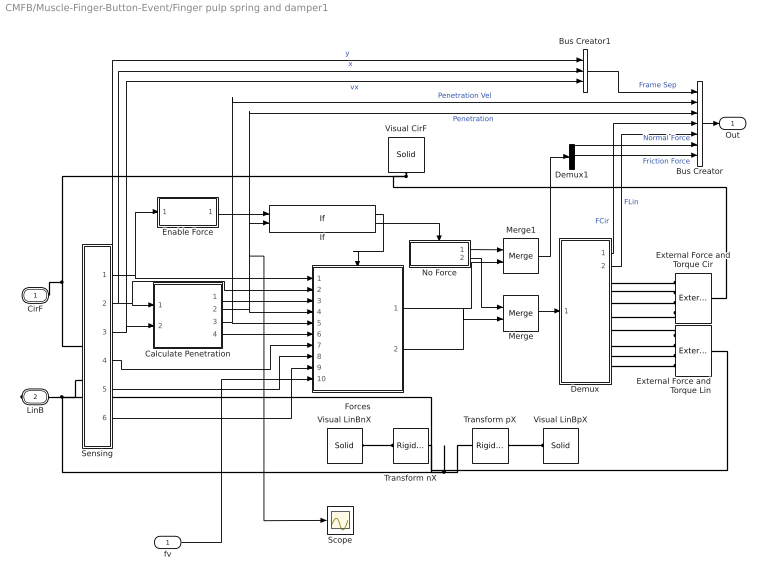
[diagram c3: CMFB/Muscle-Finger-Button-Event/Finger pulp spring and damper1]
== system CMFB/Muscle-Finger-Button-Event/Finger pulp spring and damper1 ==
  fv : Inport
  Bus Creator : BusCreator  Inputs=7
  Bus Creator1 : BusCreator  Inputs=3
  Calculate Penetration : Subsystem
  Demux : Subsystem
  Demux1 : Demux  Outputs=2
  Enable Force : Subsystem
  External Force and Torque Cir : sm_lib/Forces and Torques/External Force and Torque  ForceResolutionFrame=AttachedFrame  EnableForceX=on  EnableForceY=on  EnableForceZ=on  EnableForce=off  TorqueResolutionFrame=AttachedFrame  EnableTorqueX=off  EnableTorqueY=off  EnableTorqueZ=on  EnableTorque=off
  External Force and Torque Lin : sm_lib/Forces and Torques/External Force and Torque  ForceResolutionFrame=AttachedFrame  EnableForceX=on  EnableForceY=on  EnableForceZ=on  EnableForce=off  TorqueResolutionFrame=AttachedFrame  EnableTorqueX=off  EnableTorqueY=off  EnableTorqueZ=on  EnableTorque=off
  Forces : Subsystem
  If : If  NumInputs=2  IfExpression=(u1 > 0)
  Merge : Merge  InitialOutput=0  InputPortOffsets=0
  Merge1 : Merge  InitialOutput=0  InputPortOffsets=0
  No Force : Subsystem
  Scope : Scope
  Sensing : Subsystem
  Transform nX : sm_lib/Frames and Transforms/Rigid Transform  TranslationMethod=StandardAxis  TranslationStandardOffset=line_depth-vis_len_linBx/2  TranslationLengthUnit=m  TranslationStandardAxis=-X  TranslationCartesianOffset=[0 0 0]  TranslationROffset=0  TranslationROffsetUnits=m  TranslationZOffset=0  TranslationZOffsetUnits=m  TranslationThetaOffset=0  TranslationThetaOffsetUnits=deg  RotationMethod=None  RotationAngleUnits=deg  RotationStandardAxis=+Z  RotationAngle=0.0  RotationArbitraryAxis=[0 0 1]  FollAlignAxisA=+X  BaseAlignAxisA=+Y  FollAlignAxisB=+Y  BaseAlignAxisB=+Z  RotationSequenceAxes=FollowerAxes  RotationSequence=XYX  RotationSequenceAngles=[0 0 0]  RotationSequenceAnglesUnits=deg  RotationMatrix=[1 0 0; 0 1 0; 0 0 1]
  Transform pX : sm_lib/Frames and Transforms/Rigid Transform  TranslationMethod=StandardAxis  TranslationStandardOffset=line_depth-vis_len_linBx/2  TranslationLengthUnit=m  TranslationStandardAxis=+X  TranslationCartesianOffset=[0 0 0]  TranslationROffset=0  TranslationROffsetUnits=m  TranslationZOffset=0  TranslationZOffsetUnits=m  TranslationThetaOffset=0  TranslationThetaOffsetUnits=deg  RotationMethod=None  RotationAngleUnits=deg  RotationStandardAxis=+Z  RotationAngle=0.0  RotationArbitraryAxis=[0 0 1]  FollAlignAxisA=+X  BaseAlignAxisA=+Y  FollAlignAxisB=+Y  BaseAlignAxisB=+Z  RotationSequenceAxes=FollowerAxes  RotationSequence=XYX  RotationSequenceAngles=[0 0 0]  RotationSequenceAnglesUnits=deg  RotationMatrix=[1 0 0; 0 1 0; 0 0 1]
  Visual CirF : sm_lib/Body Elements/Solid  InertiaType=CalculateFromGeometry  Mass=1  MassUnits=kg  CenterOfMass=[0 0 0]  CenterOfMassUnits=m  MomentsOfInertia=[1 1 1]  MomentsOfInertiaUnits=kg*m^2  ProductsOfInertia=[0 0 0]  ProductsOfInertiaUnits=kg*m^2  DensityBased=on  Density=0  DensityUnits=kg/(m^3)  DoExposeReferenceFrame=on  SerializedFrames=<Frames/>  GraphicType=FromGeometry  MarkerShape=Sphere  MarkerSize=10  GraphicVisPropType=SimpleVisualProperties  GraphicDiffuseColor=vis_clr  GraphicSpecularColor=[0.5 0.5 0.5 1.0]  GraphicAmbientColor=[0.15 0.15 0.15 1.0]  GraphicEmissiveColor=[0.0 0.0 0.0 1.0]  GraphicShininess=75  GraphicOpacity=vis_opc*vis_opc_en  GeometryShape=GeneralExtrusion  RectangleSize=[1 1]  RectangleSizeUnits=m  BrickDimensions=[1 1 1]  BrickDimensionUnits=m  CylinderRadius=1  CylinderRadiusUnits=m  CylinderLength=1  CylinderLengthUnits=m  SphereRadius=1  SphereRadiusUnits=m  EllipsoidRadii=[1 1 1]  EllipsoidRadiiUnits=m  ExtrusionCrossSection=Extr_Data_Ring(circle_rad,circle_rad-vis_len_cirFx,0,360)  ExtrusionCrossSectionUnits=m  ExtrusionLength=vis_len_cirFz  ExtrusionLengthUnits=m  PolygonNumSides=3  PolygonOuterRadius=1  PolygonOuterRadiusUnits=m  ExtGeomFileType=STEP  ExtGeomFileUnits=m  RevolutionCrossSection=[1 1; 1 -1; 2 -1; 2 1]  RevolutionCrossSectionUnits=m  RevolutionExtent=Full  RevolutionAngle=180  RevolutionAngleUnits=deg
  Visual LinBnX : sm_lib/Body Elements/Solid  InertiaType=CalculateFromGeometry  Mass=1  MassUnits=kg  CenterOfMass=[0 0 0]  CenterOfMassUnits=m  MomentsOfInertia=[1 1 1]  MomentsOfInertiaUnits=kg*m^2  ProductsOfInertia=[0 0 0]  ProductsOfInertiaUnits=kg*m^2  DensityBased=on  Density=0  DensityUnits=kg/(m^3)  DoExposeReferenceFrame=on  SerializedFrames=<Frames/>  GraphicType=FromGeometry  MarkerShape=Sphere  MarkerSize=10  GraphicVisPropType=SimpleVisualProperties  GraphicDiffuseColor=vis_clr  GraphicSpecularColor=[0.5 0.5 0.5 1.0]  GraphicAmbientColor=[0.15 0.15 0.15 1.0]  GraphicEmissiveColor=[0.0 0.0 0.0 1.0]  GraphicShininess=75  GraphicOpacity=vis_opc*vis_opc_en  GeometryShape=Brick  RectangleSize=[1 1]  RectangleSizeUnits=m  BrickDimensions=[vis_len_linBx line_length vis_len_linBz]  BrickDimensionUnits=m  CylinderRadius=1  CylinderRadiusUnits=m  CylinderLength=1  CylinderLengthUnits=m  SphereRadius=1  SphereRadiusUnits=m  EllipsoidRadii=[1 1 1]  EllipsoidRadiiUnits=m  ExtrusionCrossSection=[1 1; -1 1; -1 -1; 1 -1]  ExtrusionCrossSectionUnits=m  ExtrusionLength=1  ExtrusionLengthUnits=m  PolygonNumSides=3  PolygonOuterRadius=1  PolygonOuterRadiusUnits=m  ExtGeomFileType=STEP  ExtGeomFileUnits=m  RevolutionCrossSection=[1 1; 1 -1; 2 -1; 2 1]  RevolutionCrossSectionUnits=m  RevolutionExtent=Full  RevolutionAngle=180  RevolutionAngleUnits=deg
  Visual LinBpX : sm_lib/Body Elements/Solid  InertiaType=CalculateFromGeometry  Mass=1  MassUnits=kg  CenterOfMass=[0 0 0]  CenterOfMassUnits=m  MomentsOfInertia=[1 1 1]  MomentsOfInertiaUnits=kg*m^2  ProductsOfInertia=[0 0 0]  ProductsOfInertiaUnits=kg*m^2  DensityBased=on  Density=0  DensityUnits=kg/(m^3)  DoExposeReferenceFrame=on  SerializedFrames=<Frames/>  GraphicType=FromGeometry  MarkerShape=Sphere  MarkerSize=10  GraphicVisPropType=SimpleVisualProperties  GraphicDiffuseColor=vis_clr  GraphicSpecularColor=[0.5 0.5 0.5 1.0]  GraphicAmbientColor=[0.15 0.15 0.15 1.0]  GraphicEmissiveColor=[0.0 0.0 0.0 1.0]  GraphicShininess=75  GraphicOpacity=vis_opc*vis_opc_en  GeometryShape=Brick  RectangleSize=[1 1]  RectangleSizeUnits=m  BrickDimensions=[vis_len_linBx line_length vis_len_linBz]  BrickDimensionUnits=m  CylinderRadius=1  CylinderRadiusUnits=m  CylinderLength=1  CylinderLengthUnits=m  SphereRadius=1  SphereRadiusUnits=m  EllipsoidRadii=[1 1 1]  EllipsoidRadiiUnits=m  ExtrusionCrossSection=[1 1; -1 1; -1 -1; 1 -1]  ExtrusionCrossSectionUnits=m  ExtrusionLength=1  ExtrusionLengthUnits=m  PolygonNumSides=3  PolygonOuterRadius=1  PolygonOuterRadiusUnits=m  ExtGeomFileType=STEP  ExtGeomFileUnits=m  RevolutionCrossSection=[1 1; 1 -1; 2 -1; 2 1]  RevolutionCrossSectionUnits=m  RevolutionExtent=Full  RevolutionAngle=180  RevolutionAngleUnits=deg
  CirF : PMIOPort  Tag=PMCPort  Port=1  Side=Left
  LinB : PMIOPort  Tag=PMCPort  Port=2  Side=Right
  Out : Outport
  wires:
  Merge1/1 -> Demux1/1
  Forces/1(Fnf) -> Merge1/2
  No Force/1(Fnf) -> Merge1/1
  Demux1/2 -> Bus Creator/7  "Friction Force"
  Demux1/1 -> Bus Creator/6  "Normal Force"
  Bus Creator1/1 -> Bus Creator/1  "Frame Sep"
  Bus Creator/1 -> Out/1
  Demux/1(FCir) -> Bus Creator/4  "FCir"
  Demux/2(FLin) -> Bus Creator/5  "FLin"
  Sensing/2(x) -> Bus Creator1/2, Forces/2(X Sep), Calculate Penetration/1(x)  "x"
  Sensing/3(vx) -> Calculate Penetration/2(vx), Bus Creator1/3  "vx"
  Calculate Penetration/4(Vel Sign) -> Forces/6(Vel_Cmp)
  Calculate Penetration/1(Pos Sign) -> Forces/3(Pos Cmp)
  Sensing/1(y) -> Bus Creator1/1, Enable Force/1(y), Forces/1(M arm)  "y"
  Calculate Penetration/2(Pen) -> Scope/1, If/2, Bus Creator/3, Forces/4(Pen)  "Penetration"
  Enable Force/1(Enable) -> If/1
  If/1 -> Forces/Action
  No Force/2(F) -> Merge/1
  If/2 -> No Force/Action
  Merge/1 -> Demux/1(F)
  Calculate Penetration/3(Pen Vel) -> Forces/5(Vel), Bus Creator/2  "Penetration Vel"
  Sensing/4(q) -> Forces/7(Unit Vector)
  Forces/2(F) -> Merge/2
  Sensing/5(vy) -> Forces/8(vy)
  Sensing/6(wz) -> Forces/9(wz)
  fv/1 -> Forces/10("finger velo ")
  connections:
  Transform nX/RConn1 -- Visual LinBnX/RConn1
  Transform pX/RConn1 -- Visual LinBpX/RConn1
  Sensing/LConn2 -- External Force and Torque Lin/RConn1 -- Transform pX/LConn1 -- Transform nX/LConn1 -- LinB/RConn1
  Visual CirF/RConn1 -- Sensing/LConn1 -- CirF/RConn1 -- External Force and Torque Cir/RConn1
  Demux/RConn1 -- External Force and Torque Cir/LConn1
  External Force and Torque Cir/LConn2 -- Demux/RConn2
  Demux/RConn3 -- External Force and Torque Cir/LConn3
  External Force and Torque Lin/LConn1 -- Demux/RConn5
  Demux/RConn6 -- External Force and Torque Lin/LConn2
  External Force and Torque Lin/LConn3 -- Demux/RConn7
  Demux/RConn8 -- External Force and Torque Lin/LConn4
  External Force and Torque Cir/LConn4 -- Demux/RConn4

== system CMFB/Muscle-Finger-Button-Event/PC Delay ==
  PS Constant Delay : fl_lib/Physical Signals/Delays/PS Constant Delay  InputHistory=0.0  DelayTime=Button.bea_delay s
  PS-Simulink Converter : nesl_utility/PS-Simulink Converter  PhysicalDomain=network_engine_domain  SubClassName=ps_output  LeftPortType=input  RightPortType=output  PseudoPeriodic=off  Frequencies=[]  Unit=1  AffineConversion=off
  Transform Sensor : sm_lib/Frames and Transforms/Transform Sensor  MeasurementFrame=World  SenseAngle=off  SenseAxis=off  SenseAngle1=off  SenseAngle2=off  SenseAngle3=off  SenseQ=off  SenseR=off  SenseOmegaX=off  SenseOmegaY=off  SenseOmegaZ=off  SenseOmega1=off  SenseOmega2=off  SenseOmega3=off  SenseQDot=off  SenseRDot=off  SenseAlphaX=off  SenseAlphaY=off  SenseAlphaZ=off  SenseAlpha1=off  SenseAlpha2=off  SenseAlpha3=off  SenseQDDot=off  SenseRDDot=off  SenseX=off  SenseY=off  SenseZ=on  SenseRad=off  SenseAzim=off  SenseDist=off  SenseInc=off  SenseXDot=off  SenseYDot=off  SenseZDot=off  SenseRadDot=off  SenseAzimDot=off  SenseDistDot=off  SenseIncDot=off  SenseXDDot=off  SenseYDDot=off  SenseZDDot=off  SenseRadDDot=off  SenseAzimDDot=off  SenseDistDDot=off  SenseIncDDot=off
  World Frame1 : sm_lib/Frames and Transforms/World Frame
  Conn1 : PMIOPort  Port=1  Side=Right
  S : Outport
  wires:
  PS-Simulink Converter/1 -> S/1
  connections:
  Transform Sensor/RConn1 -- Conn1/RConn1
  World Frame1/RConn1 -- Transform Sensor/LConn1
  PS Constant Delay/LConn1 -- Transform Sensor/RConn2
  PS-Simulink Converter/LConn1 -- PS Constant Delay/RConn1

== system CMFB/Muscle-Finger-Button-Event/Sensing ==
  Mux : Mux  Inputs=3
  PS-Simulink Converter{,1..4} (5 alike) : nesl_utility/PS-Simulink Converter  PhysicalDomain=network_engine_domain  SubClassName=ps_output  LeftPortType=input  RightPortType=output  PseudoPeriodic=off  Frequencies=[]  Unit=1  AffineConversion=off
  Terminator : Terminator
  Transform Sensor : sm_lib/Frames and Transforms/Transform Sensor  MeasurementFrame=World  SenseAngle=off  SenseAxis=off  SenseAngle1=off  SenseAngle2=off  SenseAngle3=off  SenseQ=off  SenseR=off  SenseOmegaX=off  SenseOmegaY=off  SenseOmegaZ=off  SenseOmega1=off  SenseOmega2=off  SenseOmega3=off  SenseQDot=off  SenseRDot=off  SenseAlphaX=off  SenseAlphaY=off  SenseAlphaZ=off  SenseAlpha1=off  SenseAlpha2=off  SenseAlpha3=off  SenseQDDot=off  SenseRDDot=off  SenseX=on  SenseY=on  SenseZ=on  SenseRad=off  SenseAzim=off  SenseDist=off  SenseInc=off  SenseXDot=off  SenseYDot=off  SenseZDot=on  SenseRadDot=off  SenseAzimDot=off  SenseDistDot=off  SenseIncDot=off  SenseXDDot=off  SenseYDDot=off  SenseZDDot=on  SenseRadDDot=off  SenseAzimDDot=off  SenseDistDDot=off  SenseIncDDot=off
  World Frame : sm_lib/Frames and Transforms/World Frame
  F : PMIOPort  Port=1  Side=Left
  P : Outport
  V : Outport  Port=2
  A : Outport  Port=3
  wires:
  PS-Simulink Converter/1 -> P/1, Mux/3
  PS-Simulink Converter2/1 -> Mux/1
  PS-Simulink Converter1/1 -> Mux/2
  Mux/1 -> Terminator/1
  PS-Simulink Converter3/1 -> V/1
  PS-Simulink Converter4/1 -> A/1
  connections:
  World Frame/RConn1 -- Transform Sensor/LConn1
  F/RConn1 -- Transform Sensor/RConn1
  PS-Simulink Converter/LConn1 -- Transform Sensor/RConn4
  PS-Simulink Converter1/LConn1 -- Transform Sensor/RConn3
  PS-Simulink Converter2/LConn1 -- Transform Sensor/RConn2
  PS-Simulink Converter3/LConn1 -- Transform Sensor/RConn5
  PS-Simulink Converter4/LConn1 -- Transform Sensor/RConn6

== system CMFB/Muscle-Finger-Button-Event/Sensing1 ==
  Mux : Mux  Inputs=3
  PS-Simulink Converter : nesl_utility/PS-Simulink Converter  PhysicalDomain=network_engine_domain  SubClassName=ps_output  LeftPortType=input  RightPortType=output  PseudoPeriodic=off  Frequencies=[]  Unit=1  AffineConversion=off
  PS-Simulink Converter1 : nesl_utility/PS-Simulink Converter  PhysicalDomain=network_engine_domain  SubClassName=ps_output  LeftPortType=input  RightPortType=output  PseudoPeriodic=off  Frequencies=[]  Unit=1  AffineConversion=off
  PS-Simulink Converter2 : nesl_utility/PS-Simulink Converter  PhysicalDomain=network_engine_domain  SubClassName=ps_output  LeftPortType=input  RightPortType=output  PseudoPeriodic=off  Frequencies=[]  Unit=1  AffineConversion=off
  Terminator : Terminator
  Transform Sensor : sm_lib/Frames and Transforms/Transform Sensor  MeasurementFrame=World  SenseAngle=off  SenseAxis=off  SenseAngle1=off  SenseAngle2=off  SenseAngle3=off  SenseQ=off  SenseR=off  SenseOmegaX=off  SenseOmegaY=off  SenseOmegaZ=off  SenseOmega1=off  SenseOmega2=off  SenseOmega3=off  SenseQDot=off  SenseRDot=off  SenseAlphaX=off  SenseAlphaY=off  SenseAlphaZ=off  SenseAlpha1=off  SenseAlpha2=off  SenseAlpha3=off  SenseQDDot=off  SenseRDDot=off  SenseX=on  SenseY=on  SenseZ=on  SenseRad=off  SenseAzim=off  SenseDist=off  SenseInc=off  SenseXDot=off  SenseYDot=off  SenseZDot=off  SenseRadDot=off  SenseAzimDot=off  SenseDistDot=off  SenseIncDot=off  SenseXDDot=off  SenseYDDot=off  SenseZDDot=off  SenseRadDDot=off  SenseAzimDDot=off  SenseDistDDot=off  SenseIncDDot=off
  World Frame : sm_lib/Frames and Transforms/World Frame
  F : PMIOPort  Port=1  Side=Left
  S : Outport
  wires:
  PS-Simulink Converter/1 -> S/1, Mux/3
  PS-Simulink Converter2/1 -> Mux/1
  PS-Simulink Converter1/1 -> Mux/2
  Mux/1 -> Terminator/1
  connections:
  World Frame/RConn1 -- Transform Sensor/LConn1
  F/RConn1 -- Transform Sensor/RConn1
  PS-Simulink Converter/LConn1 -- Transform Sensor/RConn4
  PS-Simulink Converter1/LConn1 -- Transform Sensor/RConn3
  PS-Simulink Converter2/LConn1 -- Transform Sensor/RConn2
